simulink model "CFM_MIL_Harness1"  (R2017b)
settings: Solver=FixedStepDiscrete  StartTime=0.0  StopTime=14  FixedStep=0.01  RelTol=1e-3  EnableMultiTasking=on
undefined symbols (not defined in the file): sigbuilder_block
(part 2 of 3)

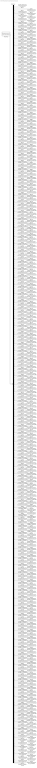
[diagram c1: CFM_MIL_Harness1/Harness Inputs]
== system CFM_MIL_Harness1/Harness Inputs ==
  Demux : Demux  Tag=STV Demux  Outputs=425
  FromWs : FromWorkspace  Tag=STV FromWs  VariableName=tuvar  SampleTime=0
  GaISP_AFEComLost_numb(1) : Outport  Tag=STV Outport
  GaISP_AFEComLost_numb(2) : Outport  Tag=STV Outport  Port=2
  GaISP_AFEComLost_numb(3) : Outport  Tag=STV Outport  Port=3
  GaISP_AFEComLost_numb(4) : Outport  Tag=STV Outport  Port=4
  GaISP_AFEComLost_numb(5) : Outport  Tag=STV Outport  Port=5
  GaISP_AFEComLost_numb(6) : Outport  Tag=STV Outport  Port=6
  GaISP_AFEComLost_numb(7) : Outport  Tag=STV Outport  Port=7
  GaISP_AFEComLost_numb(8) : Outport  Tag=STV Outport  Port=8
  GaISP_AFECellVoltUpdErr_numb(1) : Outport  Tag=STV Outport  Port=9
  GaISP_AFECellVoltUpdErr_numb(2) : Outport  Tag=STV Outport  Port=10
  GaISP_AFECellVoltUpdErr_numb(3) : Outport  Tag=STV Outport  Port=11
  GaISP_AFECellVoltUpdErr_numb(4) : Outport  Tag=STV Outport  Port=12
  GaISP_AFECellVoltUpdErr_numb(5) : Outport  Tag=STV Outport  Port=13
  GaISP_AFECellVoltUpdErr_numb(6) : Outport  Tag=STV Outport  Port=14
  GaISP_AFECellVoltUpdErr_numb(7) : Outport  Tag=STV Outport  Port=15
  GaISP_AFECellVoltUpdErr_numb(8) : Outport  Tag=STV Outport  Port=16
  GaISP_AFECellVoltUpdErr_numb(9) : Outport  Tag=STV Outport  Port=17
  GaISP_AFECellVoltUpdErr_numb(10) : Outport  Tag=STV Outport  Port=18
  GaISP_AFECellVoltUpdErr_numb(11) : Outport  Tag=STV Outport  Port=19
  GaISP_AFECellVoltUpdErr_numb(12) : Outport  Tag=STV Outport  Port=20
  GaISP_AFECellVoltUpdErr_numb(13) : Outport  Tag=STV Outport  Port=21
  GaISP_AFECellVoltUpdErr_numb(14) : Outport  Tag=STV Outport  Port=22
  GaISP_AFECellVoltUpdErr_numb(15) : Outport  Tag=STV Outport  Port=23
  GaISP_AFECellVoltUpdErr_numb(16) : Outport  Tag=STV Outport  Port=24
  GaISP_AFECellVoltUpdErr_numb(17) : Outport  Tag=STV Outport  Port=25
  GaISP_AFECellVoltUpdErr_numb(18) : Outport  Tag=STV Outport  Port=26
  GaISP_AFECellVoltUpdErr_numb(19) : Outport  Tag=STV Outport  Port=27
  GaISP_AFECellVoltUpdErr_numb(20) : Outport  Tag=STV Outport  Port=28
  GaISP_AFECellVoltUpdErr_numb(21) : Outport  Tag=STV Outport  Port=29
  GaISP_AFECellVoltUpdErr_numb(22) : Outport  Tag=STV Outport  Port=30
  GaISP_AFECellVoltUpdErr_numb(23) : Outport  Tag=STV Outport  Port=31
  GaISP_AFECellVoltUpdErr_numb(24) : Outport  Tag=STV Outport  Port=32
  GaISP_AFECellVoltUpdErr_numb(25) : Outport  Tag=STV Outport  Port=33
  GaISP_AFECellVoltUpdErr_numb(26) : Outport  Tag=STV Outport  Port=34
  GaISP_AFECellVoltUpdErr_numb(27) : Outport  Tag=STV Outport  Port=35
  GaISP_AFECellVoltUpdErr_numb(28) : Outport  Tag=STV Outport  Port=36
  GaISP_AFECellVoltUpdErr_numb(29) : Outport  Tag=STV Outport  Port=37
  GaISP_AFECellVoltUpdErr_numb(30) : Outport  Tag=STV Outport  Port=38
  GaISP_AFECellVoltUpdErr_numb(31) : Outport  Tag=STV Outport  Port=39
  GaISP_AFECellVoltUpdErr_numb(32) : Outport  Tag=STV Outport  Port=40
  GaISP_AFECellVoltUpdErr_numb(33) : Outport  Tag=STV Outport  Port=41
  GaISP_AFECellVoltUpdErr_numb(34) : Outport  Tag=STV Outport  Port=42
  GaISP_AFECellVoltUpdErr_numb(35) : Outport  Tag=STV Outport  Port=43
  GaISP_AFECellVoltUpdErr_numb(36) : Outport  Tag=STV Outport  Port=44
  GaISP_AFECellVoltUpdErr_numb(37) : Outport  Tag=STV Outport  Port=45
  GaISP_AFECellVoltUpdErr_numb(38) : Outport  Tag=STV Outport  Port=46
  GaISP_AFECellVoltUpdErr_numb(39) : Outport  Tag=STV Outport  Port=47
  GaISP_AFECellVoltUpdErr_numb(40) : Outport  Tag=STV Outport  Port=48
  GaISP_AFECellVoltUpdErr_numb(41) : Outport  Tag=STV Outport  Port=49
  GaISP_AFECellVoltUpdErr_numb(42) : Outport  Tag=STV Outport  Port=50
  GaISP_AFECellVoltUpdErr_numb(43) : Outport  Tag=STV Outport  Port=51
  GaISP_AFECellVoltUpdErr_numb(44) : Outport  Tag=STV Outport  Port=52
  GaISP_AFECellVoltUpdErr_numb(45) : Outport  Tag=STV Outport  Port=53
  GaISP_AFECellVoltUpdErr_numb(46) : Outport  Tag=STV Outport  Port=54
  GaISP_AFECellVoltUpdErr_numb(47) : Outport  Tag=STV Outport  Port=55
  GaISP_AFECellVoltUpdErr_numb(48) : Outport  Tag=STV Outport  Port=56
  GaISP_AFECellVoltUpdErr_numb(49) : Outport  Tag=STV Outport  Port=57
  GaISP_AFECellVoltUpdErr_numb(50) : Outport  Tag=STV Outport  Port=58
  GaISP_AFECellVoltUpdErr_numb(51) : Outport  Tag=STV Outport  Port=59
  GaISP_AFECellVoltUpdErr_numb(52) : Outport  Tag=STV Outport  Port=60
  GaISP_AFECellVoltUpdErr_numb(53) : Outport  Tag=STV Outport  Port=61
  GaISP_AFECellVoltUpdErr_numb(54) : Outport  Tag=STV Outport  Port=62
  GaISP_AFECellVoltUpdErr_numb(55) : Outport  Tag=STV Outport  Port=63
  GaISP_AFECellVoltUpdErr_numb(56) : Outport  Tag=STV Outport  Port=64
  GaISP_AFECellVoltUpdErr_numb(57) : Outport  Tag=STV Outport  Port=65
  GaISP_AFECellVoltUpdErr_numb(58) : Outport  Tag=STV Outport  Port=66
  GaISP_AFECellVoltUpdErr_numb(59) : Outport  Tag=STV Outport  Port=67
  GaISP_AFECellVoltUpdErr_numb(60) : Outport  Tag=STV Outport  Port=68
  GaISP_AFECellVoltUpdErr_numb(61) : Outport  Tag=STV Outport  Port=69
  GaISP_AFECellVoltUpdErr_numb(62) : Outport  Tag=STV Outport  Port=70
  GaISP_AFECellVoltUpdErr_numb(63) : Outport  Tag=STV Outport  Port=71
  GaISP_AFECellVoltUpdErr_numb(64) : Outport  Tag=STV Outport  Port=72
  GaISP_AFECellVoltUpdErr_numb(65) : Outport  Tag=STV Outport  Port=73
  GaISP_AFECellVoltUpdErr_numb(66) : Outport  Tag=STV Outport  Port=74
  GaISP_AFECellVoltUpdErr_numb(67) : Outport  Tag=STV Outport  Port=75
  GaISP_AFECellVoltUpdErr_numb(68) : Outport  Tag=STV Outport  Port=76
  GaISP_AFECellVoltUpdErr_numb(69) : Outport  Tag=STV Outport  Port=77
  GaISP_AFECellVoltUpdErr_numb(70) : Outport  Tag=STV Outport  Port=78
  GaISP_AFECellVoltUpdErr_numb(71) : Outport  Tag=STV Outport  Port=79
  GaISP_AFECellVoltUpdErr_numb(72) : Outport  Tag=STV Outport  Port=80
  GaISP_AFECellVoltUpdErr_numb(73) : Outport  Tag=STV Outport  Port=81
  GaISP_AFECellVoltUpdErr_numb(74) : Outport  Tag=STV Outport  Port=82
  GaISP_AFECellVoltUpdErr_numb(75) : Outport  Tag=STV Outport  Port=83
  GaISP_AFECellVoltUpdErr_numb(76) : Outport  Tag=STV Outport  Port=84
  GaISP_AFECellVoltUpdErr_numb(77) : Outport  Tag=STV Outport  Port=85
  GaISP_AFECellVoltUpdErr_numb(78) : Outport  Tag=STV Outport  Port=86
  GaISP_AFECellVoltUpdErr_numb(79) : Outport  Tag=STV Outport  Port=87
  GaISP_AFECellVoltUpdErr_numb(80) : Outport  Tag=STV Outport  Port=88
  GaISP_AFECellVoltUpdErr_numb(81) : Outport  Tag=STV Outport  Port=89
  GaISP_AFECellVoltUpdErr_numb(82) : Outport  Tag=STV Outport  Port=90
  GaISP_AFECellVoltUpdErr_numb(83) : Outport  Tag=STV Outport  Port=91
  GaISP_AFECellVoltUpdErr_numb(84) : Outport  Tag=STV Outport  Port=92
  GaISP_AFECellVoltUpdErr_numb(85) : Outport  Tag=STV Outport  Port=93
  GaISP_AFECellVoltUpdErr_numb(86) : Outport  Tag=STV Outport  Port=94
  GaISP_AFECellVoltUpdErr_numb(87) : Outport  Tag=STV Outport  Port=95
  GaISP_AFECellVoltUpdErr_numb(88) : Outport  Tag=STV Outport  Port=96
  GaISP_AFECellVoltUpdErr_numb(89) : Outport  Tag=STV Outport  Port=97
  GaISP_AFECellVoltUpdErr_numb(90) : Outport  Tag=STV Outport  Port=98
  GaISP_AFECellVoltUpdErr_numb(91) : Outport  Tag=STV Outport  Port=99
  GaISP_AFECellVoltUpdErr_numb(92) : Outport  Tag=STV Outport  Port=100
  GaISP_AFECellVoltUpdErr_numb(93) : Outport  Tag=STV Outport  Port=101
  GaISP_AFECellVoltUpdErr_numb(94) : Outport  Tag=STV Outport  Port=102
  GaISP_AFECellVoltUpdErr_numb(95) : Outport  Tag=STV Outport  Port=103
  GaISP_AFECellVoltUpdErr_numb(96) : Outport  Tag=STV Outport  Port=104
  GaISP_AFECellVoltUpdErr_numb(97) : Outport  Tag=STV Outport  Port=105
  GaISP_AFECellVoltUpdErr_numb(98) : Outport  Tag=STV Outport  Port=106
  GaISP_AFECellVoltUpdErr_numb(99) : Outport  Tag=STV Outport  Port=107
  GaISP_AFECellVoltUpdErr_numb(100) : Outport  Tag=STV Outport  Port=108
  GaISP_AFECellVoltUpdErr_numb(101) : Outport  Tag=STV Outport  Port=109
  GaISP_AFECellVoltUpdErr_numb(102) : Outport  Tag=STV Outport  Port=110
  GaISP_AFECellVoltUpdErr_numb(103) : Outport  Tag=STV Outport  Port=111
  GaISP_AFECellVoltUpdErr_numb(104) : Outport  Tag=STV Outport  Port=112
  GaISP_AFECellVoltUpdErr_numb(105) : Outport  Tag=STV Outport  Port=113
  GaISP_AFECellVoltUpdErr_numb(106) : Outport  Tag=STV Outport  Port=114
  GaISP_AFECellVoltUpdErr_numb(107) : Outport  Tag=STV Outport  Port=115
  GaISP_AFECellVoltUpdErr_numb(108) : Outport  Tag=STV Outport  Port=116
  GaISP_AFECellVoltUpdErr_numb(109) : Outport  Tag=STV Outport  Port=117
  GaISP_AFECellVoltUpdErr_numb(110) : Outport  Tag=STV Outport  Port=118
  GaISP_AFECellVoltUpdErr_numb(111) : Outport  Tag=STV Outport  Port=119
  GaISP_AFECellVoltUpdErr_numb(112) : Outport  Tag=STV Outport  Port=120
  GaISP_AFECellTempUpdErr_numb(1) : Outport  Tag=STV Outport  Port=121
  GaISP_AFECellTempUpdErr_numb(2) : Outport  Tag=STV Outport  Port=122
  GaISP_AFECellTempUpdErr_numb(3) : Outport  Tag=STV Outport  Port=123
  GaISP_AFECellTempUpdErr_numb(4) : Outport  Tag=STV Outport  Port=124
  GaISP_AFECellTempUpdErr_numb(5) : Outport  Tag=STV Outport  Port=125
  GaISP_AFECellTempUpdErr_numb(6) : Outport  Tag=STV Outport  Port=126
  GaISP_AFECellTempUpdErr_numb(7) : Outport  Tag=STV Outport  Port=127
  GaISP_AFECellTempUpdErr_numb(8) : Outport  Tag=STV Outport  Port=128
  GaISP_AFECellTempUpdErr_numb(9) : Outport  Tag=STV Outport  Port=129
  GaISP_AFECellTempUpdErr_numb(10) : Outport  Tag=STV Outport  Port=130
  GaISP_AFECellTempUpdErr_numb(11) : Outport  Tag=STV Outport  Port=131
  GaISP_AFECellTempUpdErr_numb(12) : Outport  Tag=STV Outport  Port=132
  GaISP_AFECellTempUpdErr_numb(13) : Outport  Tag=STV Outport  Port=133
  GaISP_AFECellTempUpdErr_numb(14) : Outport  Tag=STV Outport  Port=134
  GaISP_AFECellTempUpdErr_numb(15) : Outport  Tag=STV Outport  Port=135
  GaISP_AFECellTempUpdErr_numb(16) : Outport  Tag=STV Outport  Port=136
  GaISP_AFECellTempUpdErr_numb(17) : Outport  Tag=STV Outport  Port=137
  GaISP_AFECellTempUpdErr_numb(18) : Outport  Tag=STV Outport  Port=138
  GaISP_AFECellTempUpdErr_numb(19) : Outport  Tag=STV Outport  Port=139
  GaISP_AFECellTempUpdErr_numb(20) : Outport  Tag=STV Outport  Port=140
  GaISP_AFECellTempUpdErr_numb(21) : Outport  Tag=STV Outport  Port=141
  GaISP_AFECellTempUpdErr_numb(22) : Outport  Tag=STV Outport  Port=142
  GaISP_AFECellTempUpdErr_numb(23) : Outport  Tag=STV Outport  Port=143
  GaISP_AFECellTempUpdErr_numb(24) : Outport  Tag=STV Outport  Port=144
  GaISP_AFECellTempUpdErr_numb(25) : Outport  Tag=STV Outport  Port=145
  GaISP_AFECellTempUpdErr_numb(26) : Outport  Tag=STV Outport  Port=146
  GaISP_AFECellTempUpdErr_numb(27) : Outport  Tag=STV Outport  Port=147
  GaISP_AFECellTempUpdErr_numb(28) : Outport  Tag=STV Outport  Port=148
  GaISP_AFECellTempUpdErr_numb(29) : Outport  Tag=STV Outport  Port=149
  GaISP_AFECellTempUpdErr_numb(30) : Outport  Tag=STV Outport  Port=150
  GaISP_AFECellTempUpdErr_numb(31) : Outport  Tag=STV Outport  Port=151
  GaISP_AFECellTempUpdErr_numb(32) : Outport  Tag=STV Outport  Port=152
  GaISP_AFECellTempUpdErr_numb(33) : Outport  Tag=STV Outport  Port=153
  GaISP_AFECellTempUpdErr_numb(34) : Outport  Tag=STV Outport  Port=154
  GaISP_AFECellTempUpdErr_numb(35) : Outport  Tag=STV Outport  Port=155
  GaISP_AFECellTempUpdErr_numb(36) : Outport  Tag=STV Outport  Port=156
  GaISP_AFECellTempUpdErr_numb(37) : Outport  Tag=STV Outport  Port=157
  GaISP_AFECellTempUpdErr_numb(38) : Outport  Tag=STV Outport  Port=158
  GaISP_AFECellTempUpdErr_numb(39) : Outport  Tag=STV Outport  Port=159
  GaISP_AFECellTempUpdErr_numb(40) : Outport  Tag=STV Outport  Port=160
  GaISP_AFECellTempUpdErr_numb(41) : Outport  Tag=STV Outport  Port=161
  GaISP_AFECellTempUpdErr_numb(42) : Outport  Tag=STV Outport  Port=162
  GaISP_AFECellTempUpdErr_numb(43) : Outport  Tag=STV Outport  Port=163
  GaISP_AFECellTempUpdErr_numb(44) : Outport  Tag=STV Outport  Port=164
  GaISP_AFECellTempUpdErr_numb(45) : Outport  Tag=STV Outport  Port=165
  GaISP_AFECellTempUpdErr_numb(46) : Outport  Tag=STV Outport  Port=166
  GaISP_AFECellTempUpdErr_numb(47) : Outport  Tag=STV Outport  Port=167
  GaISP_AFECellTempUpdErr_numb(48) : Outport  Tag=STV Outport  Port=168
  GaISP_AFECellVoltLineOpen_numb(1) : Outport  Tag=STV Outport  Port=169
  GaISP_AFECellVoltLineOpen_numb(2) : Outport  Tag=STV Outport  Port=170
  GaISP_AFECellVoltLineOpen_numb(3) : Outport  Tag=STV Outport  Port=171
  GaISP_AFECellVoltLineOpen_numb(4) : Outport  Tag=STV Outport  Port=172
  GaISP_AFECellVoltLineOpen_numb(5) : Outport  Tag=STV Outport  Port=173
  GaISP_AFECellVoltLineOpen_numb(6) : Outport  Tag=STV Outport  Port=174
  GaISP_AFECellVoltLineOpen_numb(7) : Outport  Tag=STV Outport  Port=175
  GaISP_AFECellVoltLineOpen_numb(8) : Outport  Tag=STV Outport  Port=176
  GaISP_AFECellVoltLineOpen_numb(9) : Outport  Tag=STV Outport  Port=177
  GaISP_AFECellVoltLineOpen_numb(10) : Outport  Tag=STV Outport  Port=178
  GaISP_AFECellVoltLineOpen_numb(11) : Outport  Tag=STV Outport  Port=179
  GaISP_AFECellVoltLineOpen_numb(12) : Outport  Tag=STV Outport  Port=180
  GaISP_AFECellVoltLineOpen_numb(13) : Outport  Tag=STV Outport  Port=181
  GaISP_AFECellVoltLineOpen_numb(14) : Outport  Tag=STV Outport  Port=182
  GaISP_AFECellVoltLineOpen_numb(15) : Outport  Tag=STV Outport  Port=183
  GaISP_AFECellVoltLineOpen_numb(16) : Outport  Tag=STV Outport  Port=184
  GaISP_AFECellVoltLineOpen_numb(17) : Outport  Tag=STV Outport  Port=185
  GaISP_AFECellVoltLineOpen_numb(18) : Outport  Tag=STV Outport  Port=186
  GaISP_AFECellVoltLineOpen_numb(19) : Outport  Tag=STV Outport  Port=187
  GaISP_AFECellVoltLineOpen_numb(20) : Outport  Tag=STV Outport  Port=188
  GaISP_AFECellVoltLineOpen_numb(21) : Outport  Tag=STV Outport  Port=189
  GaISP_AFECellVoltLineOpen_numb(22) : Outport  Tag=STV Outport  Port=190
  GaISP_AFECellVoltLineOpen_numb(23) : Outport  Tag=STV Outport  Port=191
  GaISP_AFECellVoltLineOpen_numb(24) : Outport  Tag=STV Outport  Port=192
  GaISP_AFECellVoltLineOpen_numb(25) : Outport  Tag=STV Outport  Port=193
  GaISP_AFECellVoltLineOpen_numb(26) : Outport  Tag=STV Outport  Port=194
  GaISP_AFECellVoltLineOpen_numb(27) : Outport  Tag=STV Outport  Port=195
  GaISP_AFECellVoltLineOpen_numb(28) : Outport  Tag=STV Outport  Port=196
  GaISP_AFECellVoltLineOpen_numb(29) : Outport  Tag=STV Outport  Port=197
  GaISP_AFECellVoltLineOpen_numb(30) : Outport  Tag=STV Outport  Port=198
  GaISP_AFECellVoltLineOpen_numb(31) : Outport  Tag=STV Outport  Port=199
  GaISP_AFECellVoltLineOpen_numb(32) : Outport  Tag=STV Outport  Port=200
  GaISP_AFECellVoltLineOpen_numb(33) : Outport  Tag=STV Outport  Port=201
  GaISP_AFECellVoltLineOpen_numb(34) : Outport  Tag=STV Outport  Port=202
  GaISP_AFECellVoltLineOpen_numb(35) : Outport  Tag=STV Outport  Port=203
  GaISP_AFECellVoltLineOpen_numb(36) : Outport  Tag=STV Outport  Port=204
  GaISP_AFECellVoltLineOpen_numb(37) : Outport  Tag=STV Outport  Port=205
  GaISP_AFECellVoltLineOpen_numb(38) : Outport  Tag=STV Outport  Port=206
  GaISP_AFECellVoltLineOpen_numb(39) : Outport  Tag=STV Outport  Port=207
  GaISP_AFECellVoltLineOpen_numb(40) : Outport  Tag=STV Outport  Port=208
  GaISP_AFECellVoltLineOpen_numb(41) : Outport  Tag=STV Outport  Port=209
  GaISP_AFECellVoltLineOpen_numb(42) : Outport  Tag=STV Outport  Port=210
  GaISP_AFECellVoltLineOpen_numb(43) : Outport  Tag=STV Outport  Port=211
  GaISP_AFECellVoltLineOpen_numb(44) : Outport  Tag=STV Outport  Port=212
  GaISP_AFECellVoltLineOpen_numb(45) : Outport  Tag=STV Outport  Port=213
  GaISP_AFECellVoltLineOpen_numb(46) : Outport  Tag=STV Outport  Port=214
  GaISP_AFECellVoltLineOpen_numb(47) : Outport  Tag=STV Outport  Port=215
  GaISP_AFECellVoltLineOpen_numb(48) : Outport  Tag=STV Outport  Port=216
  GaISP_AFECellVoltLineOpen_numb(49) : Outport  Tag=STV Outport  Port=217
  GaISP_AFECellVoltLineOpen_numb(50) : Outport  Tag=STV Outport  Port=218
  GaISP_AFECellVoltLineOpen_numb(51) : Outport  Tag=STV Outport  Port=219
  GaISP_AFECellVoltLineOpen_numb(52) : Outport  Tag=STV Outport  Port=220
  GaISP_AFECellVoltLineOpen_numb(53) : Outport  Tag=STV Outport  Port=221
  GaISP_AFECellVoltLineOpen_numb(54) : Outport  Tag=STV Outport  Port=222
  GaISP_AFECellVoltLineOpen_numb(55) : Outport  Tag=STV Outport  Port=223
  GaISP_AFECellVoltLineOpen_numb(56) : Outport  Tag=STV Outport  Port=224
  GaISP_AFECellVoltLineOpen_numb(57) : Outport  Tag=STV Outport  Port=225
  GaISP_AFECellVoltLineOpen_numb(58) : Outport  Tag=STV Outport  Port=226
  GaISP_AFECellVoltLineOpen_numb(59) : Outport  Tag=STV Outport  Port=227
  GaISP_AFECellVoltLineOpen_numb(60) : Outport  Tag=STV Outport  Port=228
  GaISP_AFECellVoltLineOpen_numb(61) : Outport  Tag=STV Outport  Port=229
  GaISP_AFECellVoltLineOpen_numb(62) : Outport  Tag=STV Outport  Port=230
  GaISP_AFECellVoltLineOpen_numb(63) : Outport  Tag=STV Outport  Port=231
  GaISP_AFECellVoltLineOpen_numb(64) : Outport  Tag=STV Outport  Port=232
  GaISP_AFECellVoltLineOpen_numb(65) : Outport  Tag=STV Outport  Port=233
  GaISP_AFECellVoltLineOpen_numb(66) : Outport  Tag=STV Outport  Port=234
  GaISP_AFECellVoltLineOpen_numb(67) : Outport  Tag=STV Outport  Port=235
  GaISP_AFECellVoltLineOpen_numb(68) : Outport  Tag=STV Outport  Port=236
  GaISP_AFECellVoltLineOpen_numb(69) : Outport  Tag=STV Outport  Port=237
  GaISP_AFECellVoltLineOpen_numb(70) : Outport  Tag=STV Outport  Port=238
  GaISP_AFECellVoltLineOpen_numb(71) : Outport  Tag=STV Outport  Port=239
  GaISP_AFECellVoltLineOpen_numb(72) : Outport  Tag=STV Outport  Port=240
  GaISP_AFECellVoltLineOpen_numb(73) : Outport  Tag=STV Outport  Port=241
  GaISP_AFECellVoltLineOpen_numb(74) : Outport  Tag=STV Outport  Port=242
  GaISP_AFECellVoltLineOpen_numb(75) : Outport  Tag=STV Outport  Port=243
  GaISP_AFECellVoltLineOpen_numb(76) : Outport  Tag=STV Outport  Port=244
  GaISP_AFECellVoltLineOpen_numb(77) : Outport  Tag=STV Outport  Port=245
  GaISP_AFECellVoltLineOpen_numb(78) : Outport  Tag=STV Outport  Port=246
  GaISP_AFECellVoltLineOpen_numb(79) : Outport  Tag=STV Outport  Port=247
  GaISP_AFECellVoltLineOpen_numb(80) : Outport  Tag=STV Outport  Port=248
  GaISP_AFECellVoltLineOpen_numb(81) : Outport  Tag=STV Outport  Port=249
  GaISP_AFECellVoltLineOpen_numb(82) : Outport  Tag=STV Outport  Port=250
  GaISP_AFECellVoltLineOpen_numb(83) : Outport  Tag=STV Outport  Port=251
  GaISP_AFECellVoltLineOpen_numb(84) : Outport  Tag=STV Outport  Port=252
  GaISP_AFECellVoltLineOpen_numb(85) : Outport  Tag=STV Outport  Port=253
  GaISP_AFECellVoltLineOpen_numb(86) : Outport  Tag=STV Outport  Port=254
  GaISP_AFECellVoltLineOpen_numb(87) : Outport  Tag=STV Outport  Port=255
  GaISP_AFECellVoltLineOpen_numb(88) : Outport  Tag=STV Outport  Port=256
  GaISP_AFECellVoltLineOpen_numb(89) : Outport  Tag=STV Outport  Port=257
  GaISP_AFECellVoltLineOpen_numb(90) : Outport  Tag=STV Outport  Port=258
  GaISP_AFECellVoltLineOpen_numb(91) : Outport  Tag=STV Outport  Port=259
  GaISP_AFECellVoltLineOpen_numb(92) : Outport  Tag=STV Outport  Port=260
  GaISP_AFECellVoltLineOpen_numb(93) : Outport  Tag=STV Outport  Port=261
  GaISP_AFECellVoltLineOpen_numb(94) : Outport  Tag=STV Outport  Port=262
  GaISP_AFECellVoltLineOpen_numb(95) : Outport  Tag=STV Outport  Port=263
  GaISP_AFECellVoltLineOpen_numb(96) : Outport  Tag=STV Outport  Port=264
  GaISP_AFECellVoltLineOpen_numb(97) : Outport  Tag=STV Outport  Port=265
  GaISP_AFECellVoltLineOpen_numb(98) : Outport  Tag=STV Outport  Port=266
  GaISP_AFECellVoltLineOpen_numb(99) : Outport  Tag=STV Outport  Port=267
  GaISP_AFECellVoltLineOpen_numb(100) : Outport  Tag=STV Outport  Port=268
  GaISP_AFECellVoltLineOpen_numb(101) : Outport  Tag=STV Outport  Port=269
  GaISP_AFECellVoltLineOpen_numb(102) : Outport  Tag=STV Outport  Port=270
  GaISP_AFECellVoltLineOpen_numb(103) : Outport  Tag=STV Outport  Port=271
  GaISP_AFECellVoltLineOpen_numb(104) : Outport  Tag=STV Outport  Port=272
  GaISP_AFECellVoltLineOpen_numb(105) : Outport  Tag=STV Outport  Port=273
  GaISP_AFECellVoltLineOpen_numb(106) : Outport  Tag=STV Outport  Port=274
  GaISP_AFECellVoltLineOpen_numb(107) : Outport  Tag=STV Outport  Port=275
  GaISP_AFECellVoltLineOpen_numb(108) : Outport  Tag=STV Outport  Port=276
  GaISP_AFECellVoltLineOpen_numb(109) : Outport  Tag=STV Outport  Port=277
  GaISP_AFECellVoltLineOpen_numb(110) : Outport  Tag=STV Outport  Port=278
  GaISP_AFECellVoltLineOpen_numb(111) : Outport  Tag=STV Outport  Port=279
  GaISP_AFECellVoltLineOpen_numb(112) : Outport  Tag=STV Outport  Port=280
  GaCDP_AFETempSampAbn_flg(1) : Outport  Tag=STV Outport  Port=281
  GaCDP_AFETempSampAbn_flg(2) : Outport  Tag=STV Outport  Port=282
  GaCDP_AFETempSampAbn_flg(3) : Outport  Tag=STV Outport  Port=283
  GaCDP_AFETempSampAbn_flg(4) : Outport  Tag=STV Outport  Port=284
  GaCDP_AFETempSampAbn_flg(5) : Outport  Tag=STV Outport  Port=285
  GaCDP_AFETempSampAbn_flg(6) : Outport  Tag=STV Outport  Port=286
  GaCDP_AFETempSampAbn_flg(7) : Outport  Tag=STV Outport  Port=287
  GaCDP_AFETempSampAbn_flg(8) : Outport  Tag=STV Outport  Port=288
  GaISP_AFEAdcRelatedErr_numb(1) : Outport  Tag=STV Outport  Port=289
  GaISP_AFEAdcRelatedErr_numb(2) : Outport  Tag=STV Outport  Port=290
  GaISP_AFEAdcRelatedErr_numb(3) : Outport  Tag=STV Outport  Port=291
  GaISP_AFEAdcRelatedErr_numb(4) : Outport  Tag=STV Outport  Port=292
  GaISP_AFEAdcRelatedErr_numb(5) : Outport  Tag=STV Outport  Port=293
  GaISP_AFEAdcRelatedErr_numb(6) : Outport  Tag=STV Outport  Port=294
  GaISP_AFEAdcRelatedErr_numb(7) : Outport  Tag=STV Outport  Port=295
  GaISP_AFEAdcRelatedErr_numb(8) : Outport  Tag=STV Outport  Port=296
  GaISP_AFEAdcRelatedErr_numb(9) : Outport  Tag=STV Outport  Port=297
  GaISP_AFEAdcRelatedErr_numb(10) : Outport  Tag=STV Outport  Port=298
  GaISP_AFEAdcRelatedErr_numb(11) : Outport  Tag=STV Outport  Port=299
  GaISP_AFEAdcRelatedErr_numb(12) : Outport  Tag=STV Outport  Port=300
  GaISP_AFEAdcRelatedErr_numb(13) : Outport  Tag=STV Outport  Port=301
  GaISP_AFEAdcRelatedErr_numb(14) : Outport  Tag=STV Outport  Port=302
  GaISP_AFEAdcRelatedErr_numb(15) : Outport  Tag=STV Outport  Port=303
  GaISP_AFEAdcRelatedErr_numb(16) : Outport  Tag=STV Outport  Port=304
  GaISP_AFEAdcRelatedErr_numb(17) : Outport  Tag=STV Outport  Port=305
  GaISP_AFEAdcRelatedErr_numb(18) : Outport  Tag=STV Outport  Port=306
  GaISP_AFEAdcRelatedErr_numb(19) : Outport  Tag=STV Outport  Port=307
  GaISP_AFEAdcRelatedErr_numb(20) : Outport  Tag=STV Outport  Port=308
  GaISP_AFEAdcRelatedErr_numb(21) : Outport  Tag=STV Outport  Port=309
  GaISP_AFEAdcRelatedErr_numb(22) : Outport  Tag=STV Outport  Port=310
  GaISP_AFEAdcRelatedErr_numb(23) : Outport  Tag=STV Outport  Port=311
  GaISP_AFEAdcRelatedErr_numb(24) : Outport  Tag=STV Outport  Port=312
  GaISP_AFEAdcRelatedErr_numb(25) : Outport  Tag=STV Outport  Port=313
  GaISP_AFEAdcRelatedErr_numb(26) : Outport  Tag=STV Outport  Port=314
  GaISP_AFEAdcRelatedErr_numb(27) : Outport  Tag=STV Outport  Port=315
  GaISP_AFEAdcRelatedErr_numb(28) : Outport  Tag=STV Outport  Port=316
  GaISP_AFEAdcRelatedErr_numb(29) : Outport  Tag=STV Outport  Port=317
  GaISP_AFEAdcRelatedErr_numb(30) : Outport  Tag=STV Outport  Port=318
  GaISP_AFEAdcRelatedErr_numb(31) : Outport  Tag=STV Outport  Port=319
  GaISP_AFEAdcRelatedErr_numb(32) : Outport  Tag=STV Outport  Port=320
  GaISP_AFEAdcRelatedErr_numb(33) : Outport  Tag=STV Outport  Port=321
  GaISP_AFEAdcRelatedErr_numb(34) : Outport  Tag=STV Outport  Port=322
  GaISP_AFEAdcRelatedErr_numb(35) : Outport  Tag=STV Outport  Port=323
  GaISP_AFEAdcRelatedErr_numb(36) : Outport  Tag=STV Outport  Port=324
  GaISP_AFEAdcRelatedErr_numb(37) : Outport  Tag=STV Outport  Port=325
  GaISP_AFEAdcRelatedErr_numb(38) : Outport  Tag=STV Outport  Port=326
  GaISP_AFEAdcRelatedErr_numb(39) : Outport  Tag=STV Outport  Port=327
  GaISP_AFEAdcRelatedErr_numb(40) : Outport  Tag=STV Outport  Port=328
  GaISP_AFEAdcRelatedErr_numb(41) : Outport  Tag=STV Outport  Port=329
  GaISP_AFEAdcRelatedErr_numb(42) : Outport  Tag=STV Outport  Port=330
  GaISP_AFEAdcRelatedErr_numb(43) : Outport  Tag=STV Outport  Port=331
  GaISP_AFEAdcRelatedErr_numb(44) : Outport  Tag=STV Outport  Port=332
  GaISP_AFEAdcRelatedErr_numb(45) : Outport  Tag=STV Outport  Port=333
  GaISP_AFEAdcRelatedErr_numb(46) : Outport  Tag=STV Outport  Port=334
  GaISP_AFEAdcRelatedErr_numb(47) : Outport  Tag=STV Outport  Port=335
  GaISP_AFEAdcRelatedErr_numb(48) : Outport  Tag=STV Outport  Port=336
  GaISP_AFEAdcRelatedErr_numb(49) : Outport  Tag=STV Outport  Port=337
  GaISP_AFEAdcRelatedErr_numb(50) : Outport  Tag=STV Outport  Port=338
  GaISP_AFEAdcRelatedErr_numb(51) : Outport  Tag=STV Outport  Port=339
  GaISP_AFEAdcRelatedErr_numb(52) : Outport  Tag=STV Outport  Port=340
  GaISP_AFEAdcRelatedErr_numb(53) : Outport  Tag=STV Outport  Port=341
  GaISP_AFEAdcRelatedErr_numb(54) : Outport  Tag=STV Outport  Port=342
  GaISP_AFEAdcRelatedErr_numb(55) : Outport  Tag=STV Outport  Port=343
  GaISP_AFEAdcRelatedErr_numb(56) : Outport  Tag=STV Outport  Port=344
  GaISP_AFEAdcRelatedErr_numb(57) : Outport  Tag=STV Outport  Port=345
  GaISP_AFEAdcRelatedErr_numb(58) : Outport  Tag=STV Outport  Port=346
  GaISP_AFEAdcRelatedErr_numb(59) : Outport  Tag=STV Outport  Port=347
  GaISP_AFEAdcRelatedErr_numb(60) : Outport  Tag=STV Outport  Port=348
  GaISP_AFEAdcRelatedErr_numb(61) : Outport  Tag=STV Outport  Port=349
  GaISP_AFEAdcRelatedErr_numb(62) : Outport  Tag=STV Outport  Port=350
  GaISP_AFEAdcRelatedErr_numb(63) : Outport  Tag=STV Outport  Port=351
  GaISP_AFEAdcRelatedErr_numb(64) : Outport  Tag=STV Outport  Port=352
  GaISP_AFEAdcRelatedErr_numb(65) : Outport  Tag=STV Outport  Port=353
  GaISP_AFEAdcRelatedErr_numb(66) : Outport  Tag=STV Outport  Port=354
  GaISP_AFEAdcRelatedErr_numb(67) : Outport  Tag=STV Outport  Port=355
  GaISP_AFEAdcRelatedErr_numb(68) : Outport  Tag=STV Outport  Port=356
  GaISP_AFEAdcRelatedErr_numb(69) : Outport  Tag=STV Outport  Port=357
  GaISP_AFEAdcRelatedErr_numb(70) : Outport  Tag=STV Outport  Port=358
  GaISP_AFEAdcRelatedErr_numb(71) : Outport  Tag=STV Outport  Port=359
  GaISP_AFEAdcRelatedErr_numb(72) : Outport  Tag=STV Outport  Port=360
  GaISP_AFEAdcRelatedErr_numb(73) : Outport  Tag=STV Outport  Port=361
  GaISP_AFEAdcRelatedErr_numb(74) : Outport  Tag=STV Outport  Port=362
  GaISP_AFEAdcRelatedErr_numb(75) : Outport  Tag=STV Outport  Port=363
  GaISP_AFEAdcRelatedErr_numb(76) : Outport  Tag=STV Outport  Port=364
  GaISP_AFEAdcRelatedErr_numb(77) : Outport  Tag=STV Outport  Port=365
  GaISP_AFEAdcRelatedErr_numb(78) : Outport  Tag=STV Outport  Port=366
  GaISP_AFEAdcRelatedErr_numb(79) : Outport  Tag=STV Outport  Port=367
  GaISP_AFEAdcRelatedErr_numb(80) : Outport  Tag=STV Outport  Port=368
  GaISP_AFEAdcRelatedErr_numb(81) : Outport  Tag=STV Outport  Port=369
  GaISP_AFEAdcRelatedErr_numb(82) : Outport  Tag=STV Outport  Port=370
  GaISP_AFEAdcRelatedErr_numb(83) : Outport  Tag=STV Outport  Port=371
  GaISP_AFEAdcRelatedErr_numb(84) : Outport  Tag=STV Outport  Port=372
  GaISP_AFEAdcRelatedErr_numb(85) : Outport  Tag=STV Outport  Port=373
  GaISP_AFEAdcRelatedErr_numb(86) : Outport  Tag=STV Outport  Port=374
  GaISP_AFEAdcRelatedErr_numb(87) : Outport  Tag=STV Outport  Port=375
  GaISP_AFEAdcRelatedErr_numb(88) : Outport  Tag=STV Outport  Port=376
  GaISP_AFEAdcRelatedErr_numb(89) : Outport  Tag=STV Outport  Port=377
  GaISP_AFEAdcRelatedErr_numb(90) : Outport  Tag=STV Outport  Port=378
  GaISP_AFEAdcRelatedErr_numb(91) : Outport  Tag=STV Outport  Port=379
  GaISP_AFEAdcRelatedErr_numb(92) : Outport  Tag=STV Outport  Port=380
  GaISP_AFEAdcRelatedErr_numb(93) : Outport  Tag=STV Outport  Port=381
  GaISP_AFEAdcRelatedErr_numb(94) : Outport  Tag=STV Outport  Port=382
  GaISP_AFEAdcRelatedErr_numb(95) : Outport  Tag=STV Outport  Port=383
  GaISP_AFEAdcRelatedErr_numb(96) : Outport  Tag=STV Outport  Port=384
  GaISP_AFEAdcRelatedErr_numb(97) : Outport  Tag=STV Outport  Port=385
  GaISP_AFEAdcRelatedErr_numb(98) : Outport  Tag=STV Outport  Port=386
  GaISP_AFEAdcRelatedErr_numb(99) : Outport  Tag=STV Outport  Port=387
  GaISP_AFEAdcRelatedErr_numb(100) : Outport  Tag=STV Outport  Port=388
  GaISP_AFEAdcRelatedErr_numb(101) : Outport  Tag=STV Outport  Port=389
  GaISP_AFEAdcRelatedErr_numb(102) : Outport  Tag=STV Outport  Port=390
  GaISP_AFEAdcRelatedErr_numb(103) : Outport  Tag=STV Outport  Port=391
  GaISP_AFEAdcRelatedErr_numb(104) : Outport  Tag=STV Outport  Port=392
  GaISP_AFEAdcRelatedErr_numb(105) : Outport  Tag=STV Outport  Port=393
  GaISP_AFEAdcRelatedErr_numb(106) : Outport  Tag=STV Outport  Port=394
  GaISP_AFEAdcRelatedErr_numb(107) : Outport  Tag=STV Outport  Port=395
  GaISP_AFEAdcRelatedErr_numb(108) : Outport  Tag=STV Outport  Port=396
  GaISP_AFEAdcRelatedErr_numb(109) : Outport  Tag=STV Outport  Port=397
  GaISP_AFEAdcRelatedErr_numb(110) : Outport  Tag=STV Outport  Port=398
  GaISP_AFEAdcRelatedErr_numb(111) : Outport  Tag=STV Outport  Port=399
  GaISP_AFEAdcRelatedErr_numb(112) : Outport  Tag=STV Outport  Port=400
  GaISP_AFEDiagModeExitErr_numb(1) : Outport  Tag=STV Outport  Port=401
  GaISP_AFEDiagModeExitErr_numb(2) : Outport  Tag=STV Outport  Port=402
  GaISP_AFEDiagModeExitErr_numb(3) : Outport  Tag=STV Outport  Port=403
  GaISP_AFEDiagModeExitErr_numb(4) : Outport  Tag=STV Outport  Port=404
  GaISP_AFEDiagModeExitErr_numb(5) : Outport  Tag=STV Outport  Port=405
  GaISP_AFEDiagModeExitErr_numb(6) : Outport  Tag=STV Outport  Port=406
  GaISP_AFEDiagModeExitErr_numb(7) : Outport  Tag=STV Outport  Port=407
  GaISP_AFEDiagModeExitErr_numb(8) : Outport  Tag=STV Outport  Port=408
  GaISP_AFEOtherErr_numb(1) : Outport  Tag=STV Outport  Port=409
  GaISP_AFEOtherErr_numb(2) : Outport  Tag=STV Outport  Port=410
  GaISP_AFEOtherErr_numb(3) : Outport  Tag=STV Outport  Port=411
  GaISP_AFEOtherErr_numb(4) : Outport  Tag=STV Outport  Port=412
  GaISP_AFEOtherErr_numb(5) : Outport  Tag=STV Outport  Port=413
  GaISP_AFEOtherErr_numb(6) : Outport  Tag=STV Outport  Port=414
  GaISP_AFEOtherErr_numb(7) : Outport  Tag=STV Outport  Port=415
  GaISP_AFEOtherErr_numb(8) : Outport  Tag=STV Outport  Port=416
  GaISP_AFESampleErr_numb(1) : Outport  Tag=STV Outport  Port=417
  GaISP_AFESampleErr_numb(2) : Outport  Tag=STV Outport  Port=418
  GaISP_AFESampleErr_numb(3) : Outport  Tag=STV Outport  Port=419
  GaISP_AFESampleErr_numb(4) : Outport  Tag=STV Outport  Port=420
  GaISP_AFESampleErr_numb(5) : Outport  Tag=STV Outport  Port=421
  GaISP_AFESampleErr_numb(6) : Outport  Tag=STV Outport  Port=422
  GaISP_AFESampleErr_numb(7) : Outport  Tag=STV Outport  Port=423
  GaISP_AFESampleErr_numb(8) : Outport  Tag=STV Outport  Port=424
  GeUDS_CapSel_enum : Outport  Tag=STV Outport  Port=425
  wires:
  FromWs/1 -> Demux/1
  Demux/1 -> GaISP_AFEComLost_numb(1)/1
  Demux/2 -> GaISP_AFEComLost_numb(2)/1
  Demux/3 -> GaISP_AFEComLost_numb(3)/1
  Demux/4 -> GaISP_AFEComLost_numb(4)/1
  Demux/5 -> GaISP_AFEComLost_numb(5)/1
  Demux/6 -> GaISP_AFEComLost_numb(6)/1
  Demux/7 -> GaISP_AFEComLost_numb(7)/1
  Demux/8 -> GaISP_AFEComLost_numb(8)/1
  Demux/9 -> GaISP_AFECellVoltUpdErr_numb(1)/1
  Demux/10 -> GaISP_AFECellVoltUpdErr_numb(2)/1
  Demux/11 -> GaISP_AFECellVoltUpdErr_numb(3)/1
  Demux/12 -> GaISP_AFECellVoltUpdErr_numb(4)/1
  Demux/13 -> GaISP_AFECellVoltUpdErr_numb(5)/1
  Demux/14 -> GaISP_AFECellVoltUpdErr_numb(6)/1
  Demux/15 -> GaISP_AFECellVoltUpdErr_numb(7)/1
  Demux/16 -> GaISP_AFECellVoltUpdErr_numb(8)/1
  Demux/17 -> GaISP_AFECellVoltUpdErr_numb(9)/1
  Demux/18 -> GaISP_AFECellVoltUpdErr_numb(10)/1
  Demux/19 -> GaISP_AFECellVoltUpdErr_numb(11)/1
  Demux/20 -> GaISP_AFECellVoltUpdErr_numb(12)/1
  Demux/21 -> GaISP_AFECellVoltUpdErr_numb(13)/1
  Demux/22 -> GaISP_AFECellVoltUpdErr_numb(14)/1
  Demux/23 -> GaISP_AFECellVoltUpdErr_numb(15)/1
  Demux/24 -> GaISP_AFECellVoltUpdErr_numb(16)/1
  Demux/25 -> GaISP_AFECellVoltUpdErr_numb(17)/1
  Demux/26 -> GaISP_AFECellVoltUpdErr_numb(18)/1
  Demux/27 -> GaISP_AFECellVoltUpdErr_numb(19)/1
  Demux/28 -> GaISP_AFECellVoltUpdErr_numb(20)/1
  Demux/29 -> GaISP_AFECellVoltUpdErr_numb(21)/1
  Demux/30 -> GaISP_AFECellVoltUpdErr_numb(22)/1
  Demux/31 -> GaISP_AFECellVoltUpdErr_numb(23)/1
  Demux/32 -> GaISP_AFECellVoltUpdErr_numb(24)/1
  Demux/33 -> GaISP_AFECellVoltUpdErr_numb(25)/1
  Demux/34 -> GaISP_AFECellVoltUpdErr_numb(26)/1
  Demux/35 -> GaISP_AFECellVoltUpdErr_numb(27)/1
  Demux/36 -> GaISP_AFECellVoltUpdErr_numb(28)/1
  Demux/37 -> GaISP_AFECellVoltUpdErr_numb(29)/1
  Demux/38 -> GaISP_AFECellVoltUpdErr_numb(30)/1
  Demux/39 -> GaISP_AFECellVoltUpdErr_numb(31)/1
  Demux/40 -> GaISP_AFECellVoltUpdErr_numb(32)/1
  Demux/41 -> GaISP_AFECellVoltUpdErr_numb(33)/1
  Demux/42 -> GaISP_AFECellVoltUpdErr_numb(34)/1
  Demux/43 -> GaISP_AFECellVoltUpdErr_numb(35)/1
  Demux/44 -> GaISP_AFECellVoltUpdErr_numb(36)/1
  Demux/45 -> GaISP_AFECellVoltUpdErr_numb(37)/1
  Demux/46 -> GaISP_AFECellVoltUpdErr_numb(38)/1
  Demux/47 -> GaISP_AFECellVoltUpdErr_numb(39)/1
  Demux/48 -> GaISP_AFECellVoltUpdErr_numb(40)/1
  Demux/49 -> GaISP_AFECellVoltUpdErr_numb(41)/1
  Demux/50 -> GaISP_AFECellVoltUpdErr_numb(42)/1
  Demux/51 -> GaISP_AFECellVoltUpdErr_numb(43)/1
  Demux/52 -> GaISP_AFECellVoltUpdErr_numb(44)/1
  Demux/53 -> GaISP_AFECellVoltUpdErr_numb(45)/1
  Demux/54 -> GaISP_AFECellVoltUpdErr_numb(46)/1
  Demux/55 -> GaISP_AFECellVoltUpdErr_numb(47)/1
  Demux/56 -> GaISP_AFECellVoltUpdErr_numb(48)/1
  Demux/57 -> GaISP_AFECellVoltUpdErr_numb(49)/1
  Demux/58 -> GaISP_AFECellVoltUpdErr_numb(50)/1
  Demux/59 -> GaISP_AFECellVoltUpdErr_numb(51)/1
  Demux/60 -> GaISP_AFECellVoltUpdErr_numb(52)/1
  Demux/61 -> GaISP_AFECellVoltUpdErr_numb(53)/1
  Demux/62 -> GaISP_AFECellVoltUpdErr_numb(54)/1
  Demux/63 -> GaISP_AFECellVoltUpdErr_numb(55)/1
  Demux/64 -> GaISP_AFECellVoltUpdErr_numb(56)/1
  Demux/65 -> GaISP_AFECellVoltUpdErr_numb(57)/1
  Demux/66 -> GaISP_AFECellVoltUpdErr_numb(58)/1
  Demux/67 -> GaISP_AFECellVoltUpdErr_numb(59)/1
  Demux/68 -> GaISP_AFECellVoltUpdErr_numb(60)/1
  Demux/69 -> GaISP_AFECellVoltUpdErr_numb(61)/1
  Demux/70 -> GaISP_AFECellVoltUpdErr_numb(62)/1
  Demux/71 -> GaISP_AFECellVoltUpdErr_numb(63)/1
  Demux/72 -> GaISP_AFECellVoltUpdErr_numb(64)/1
  Demux/73 -> GaISP_AFECellVoltUpdErr_numb(65)/1
  Demux/74 -> GaISP_AFECellVoltUpdErr_numb(66)/1
  Demux/75 -> GaISP_AFECellVoltUpdErr_numb(67)/1
  Demux/76 -> GaISP_AFECellVoltUpdErr_numb(68)/1
  Demux/77 -> GaISP_AFECellVoltUpdErr_numb(69)/1
  Demux/78 -> GaISP_AFECellVoltUpdErr_numb(70)/1
  Demux/79 -> GaISP_AFECellVoltUpdErr_numb(71)/1
  Demux/80 -> GaISP_AFECellVoltUpdErr_numb(72)/1
  Demux/81 -> GaISP_AFECellVoltUpdErr_numb(73)/1
  Demux/82 -> GaISP_AFECellVoltUpdErr_numb(74)/1
  Demux/83 -> GaISP_AFECellVoltUpdErr_numb(75)/1
  Demux/84 -> GaISP_AFECellVoltUpdErr_numb(76)/1
  Demux/85 -> GaISP_AFECellVoltUpdErr_numb(77)/1
  Demux/86 -> GaISP_AFECellVoltUpdErr_numb(78)/1
  Demux/87 -> GaISP_AFECellVoltUpdErr_numb(79)/1
  Demux/88 -> GaISP_AFECellVoltUpdErr_numb(80)/1
  Demux/89 -> GaISP_AFECellVoltUpdErr_numb(81)/1
  Demux/90 -> GaISP_AFECellVoltUpdErr_numb(82)/1
  Demux/91 -> GaISP_AFECellVoltUpdErr_numb(83)/1
  Demux/92 -> GaISP_AFECellVoltUpdErr_numb(84)/1
  Demux/93 -> GaISP_AFECellVoltUpdErr_numb(85)/1
  Demux/94 -> GaISP_AFECellVoltUpdErr_numb(86)/1
  Demux/95 -> GaISP_AFECellVoltUpdErr_numb(87)/1
  Demux/96 -> GaISP_AFECellVoltUpdErr_numb(88)/1
  Demux/97 -> GaISP_AFECellVoltUpdErr_numb(89)/1
  Demux/98 -> GaISP_AFECellVoltUpdErr_numb(90)/1
  Demux/99 -> GaISP_AFECellVoltUpdErr_numb(91)/1
  Demux/100 -> GaISP_AFECellVoltUpdErr_numb(92)/1
  Demux/101 -> GaISP_AFECellVoltUpdErr_numb(93)/1
  Demux/102 -> GaISP_AFECellVoltUpdErr_numb(94)/1
  Demux/103 -> GaISP_AFECellVoltUpdErr_numb(95)/1
  Demux/104 -> GaISP_AFECellVoltUpdErr_numb(96)/1
  Demux/105 -> GaISP_AFECellVoltUpdErr_numb(97)/1
  Demux/106 -> GaISP_AFECellVoltUpdErr_numb(98)/1
  Demux/107 -> GaISP_AFECellVoltUpdErr_numb(99)/1
  Demux/108 -> GaISP_AFECellVoltUpdErr_numb(100)/1
  Demux/109 -> GaISP_AFECellVoltUpdErr_numb(101)/1
  Demux/110 -> GaISP_AFECellVoltUpdErr_numb(102)/1
  Demux/111 -> GaISP_AFECellVoltUpdErr_numb(103)/1
  Demux/112 -> GaISP_AFECellVoltUpdErr_numb(104)/1
  Demux/113 -> GaISP_AFECellVoltUpdErr_numb(105)/1
  Demux/114 -> GaISP_AFECellVoltUpdErr_numb(106)/1
  Demux/115 -> GaISP_AFECellVoltUpdErr_numb(107)/1
  Demux/116 -> GaISP_AFECellVoltUpdErr_numb(108)/1
  Demux/117 -> GaISP_AFECellVoltUpdErr_numb(109)/1
  Demux/118 -> GaISP_AFECellVoltUpdErr_numb(110)/1
  Demux/119 -> GaISP_AFECellVoltUpdErr_numb(111)/1
  Demux/120 -> GaISP_AFECellVoltUpdErr_numb(112)/1
  Demux/121 -> GaISP_AFECellTempUpdErr_numb(1)/1
  Demux/122 -> GaISP_AFECellTempUpdErr_numb(2)/1
  Demux/123 -> GaISP_AFECellTempUpdErr_numb(3)/1
  Demux/124 -> GaISP_AFECellTempUpdErr_numb(4)/1
  Demux/125 -> GaISP_AFECellTempUpdErr_numb(5)/1
  Demux/126 -> GaISP_AFECellTempUpdErr_numb(6)/1
  Demux/127 -> GaISP_AFECellTempUpdErr_numb(7)/1
  Demux/128 -> GaISP_AFECellTempUpdErr_numb(8)/1
  Demux/129 -> GaISP_AFECellTempUpdErr_numb(9)/1
  Demux/130 -> GaISP_AFECellTempUpdErr_numb(10)/1
  Demux/131 -> GaISP_AFECellTempUpdErr_numb(11)/1
  Demux/132 -> GaISP_AFECellTempUpdErr_numb(12)/1
  Demux/133 -> GaISP_AFECellTempUpdErr_numb(13)/1
  Demux/134 -> GaISP_AFECellTempUpdErr_numb(14)/1
  Demux/135 -> GaISP_AFECellTempUpdErr_numb(15)/1
  Demux/136 -> GaISP_AFECellTempUpdErr_numb(16)/1
  Demux/137 -> GaISP_AFECellTempUpdErr_numb(17)/1
  Demux/138 -> GaISP_AFECellTempUpdErr_numb(18)/1
  Demux/139 -> GaISP_AFECellTempUpdErr_numb(19)/1
  Demux/140 -> GaISP_AFECellTempUpdErr_numb(20)/1
  Demux/141 -> GaISP_AFECellTempUpdErr_numb(21)/1
  Demux/142 -> GaISP_AFECellTempUpdErr_numb(22)/1
  Demux/143 -> GaISP_AFECellTempUpdErr_numb(23)/1
  Demux/144 -> GaISP_AFECellTempUpdErr_numb(24)/1
  Demux/145 -> GaISP_AFECellTempUpdErr_numb(25)/1
  Demux/146 -> GaISP_AFECellTempUpdErr_numb(26)/1
  Demux/147 -> GaISP_AFECellTempUpdErr_numb(27)/1
  Demux/148 -> GaISP_AFECellTempUpdErr_numb(28)/1
  Demux/149 -> GaISP_AFECellTempUpdErr_numb(29)/1
  Demux/150 -> GaISP_AFECellTempUpdErr_numb(30)/1
  Demux/151 -> GaISP_AFECellTempUpdErr_numb(31)/1
  Demux/152 -> GaISP_AFECellTempUpdErr_numb(32)/1
  Demux/153 -> GaISP_AFECellTempUpdErr_numb(33)/1
  Demux/154 -> GaISP_AFECellTempUpdErr_numb(34)/1
  Demux/155 -> GaISP_AFECellTempUpdErr_numb(35)/1
  Demux/156 -> GaISP_AFECellTempUpdErr_numb(36)/1
  Demux/157 -> GaISP_AFECellTempUpdErr_numb(37)/1
  Demux/158 -> GaISP_AFECellTempUpdErr_numb(38)/1
  Demux/159 -> GaISP_AFECellTempUpdErr_numb(39)/1
  Demux/160 -> GaISP_AFECellTempUpdErr_numb(40)/1
  Demux/161 -> GaISP_AFECellTempUpdErr_numb(41)/1
  Demux/162 -> GaISP_AFECellTempUpdErr_numb(42)/1
  Demux/163 -> GaISP_AFECellTempUpdErr_numb(43)/1
  Demux/164 -> GaISP_AFECellTempUpdErr_numb(44)/1
  Demux/165 -> GaISP_AFECellTempUpdErr_numb(45)/1
  Demux/166 -> GaISP_AFECellTempUpdErr_numb(46)/1
  Demux/167 -> GaISP_AFECellTempUpdErr_numb(47)/1
  Demux/168 -> GaISP_AFECellTempUpdErr_numb(48)/1
  Demux/169 -> GaISP_AFECellVoltLineOpen_numb(1)/1
  Demux/170 -> GaISP_AFECellVoltLineOpen_numb(2)/1
  Demux/171 -> GaISP_AFECellVoltLineOpen_numb(3)/1
  Demux/172 -> GaISP_AFECellVoltLineOpen_numb(4)/1
  Demux/173 -> GaISP_AFECellVoltLineOpen_numb(5)/1
  Demux/174 -> GaISP_AFECellVoltLineOpen_numb(6)/1
  Demux/175 -> GaISP_AFECellVoltLineOpen_numb(7)/1
  Demux/176 -> GaISP_AFECellVoltLineOpen_numb(8)/1
  Demux/177 -> GaISP_AFECellVoltLineOpen_numb(9)/1
  Demux/178 -> GaISP_AFECellVoltLineOpen_numb(10)/1
  Demux/179 -> GaISP_AFECellVoltLineOpen_numb(11)/1
  Demux/180 -> GaISP_AFECellVoltLineOpen_numb(12)/1
  Demux/181 -> GaISP_AFECellVoltLineOpen_numb(13)/1
  Demux/182 -> GaISP_AFECellVoltLineOpen_numb(14)/1
  Demux/183 -> GaISP_AFECellVoltLineOpen_numb(15)/1
  Demux/184 -> GaISP_AFECellVoltLineOpen_numb(16)/1
  Demux/185 -> GaISP_AFECellVoltLineOpen_numb(17)/1
  Demux/186 -> GaISP_AFECellVoltLineOpen_numb(18)/1
  Demux/187 -> GaISP_AFECellVoltLineOpen_numb(19)/1
  Demux/188 -> GaISP_AFECellVoltLineOpen_numb(20)/1
  Demux/189 -> GaISP_AFECellVoltLineOpen_numb(21)/1
  Demux/190 -> GaISP_AFECellVoltLineOpen_numb(22)/1
  Demux/191 -> GaISP_AFECellVoltLineOpen_numb(23)/1
  Demux/192 -> GaISP_AFECellVoltLineOpen_numb(24)/1
  Demux/193 -> GaISP_AFECellVoltLineOpen_numb(25)/1
  Demux/194 -> GaISP_AFECellVoltLineOpen_numb(26)/1
  Demux/195 -> GaISP_AFECellVoltLineOpen_numb(27)/1
  Demux/196 -> GaISP_AFECellVoltLineOpen_numb(28)/1
  Demux/197 -> GaISP_AFECellVoltLineOpen_numb(29)/1
  Demux/198 -> GaISP_AFECellVoltLineOpen_numb(30)/1
  Demux/199 -> GaISP_AFECellVoltLineOpen_numb(31)/1
  Demux/200 -> GaISP_AFECellVoltLineOpen_numb(32)/1
  Demux/201 -> GaISP_AFECellVoltLineOpen_numb(33)/1
  Demux/202 -> GaISP_AFECellVoltLineOpen_numb(34)/1
  Demux/203 -> GaISP_AFECellVoltLineOpen_numb(35)/1
  Demux/204 -> GaISP_AFECellVoltLineOpen_numb(36)/1
  Demux/205 -> GaISP_AFECellVoltLineOpen_numb(37)/1
  Demux/206 -> GaISP_AFECellVoltLineOpen_numb(38)/1
  Demux/207 -> GaISP_AFECellVoltLineOpen_numb(39)/1
  Demux/208 -> GaISP_AFECellVoltLineOpen_numb(40)/1
  Demux/209 -> GaISP_AFECellVoltLineOpen_numb(41)/1
  Demux/210 -> GaISP_AFECellVoltLineOpen_numb(42)/1
  Demux/211 -> GaISP_AFECellVoltLineOpen_numb(43)/1
  Demux/212 -> GaISP_AFECellVoltLineOpen_numb(44)/1
  Demux/213 -> GaISP_AFECellVoltLineOpen_numb(45)/1
  Demux/214 -> GaISP_AFECellVoltLineOpen_numb(46)/1
  Demux/215 -> GaISP_AFECellVoltLineOpen_numb(47)/1
  Demux/216 -> GaISP_AFECellVoltLineOpen_numb(48)/1
  Demux/217 -> GaISP_AFECellVoltLineOpen_numb(49)/1
  Demux/218 -> GaISP_AFECellVoltLineOpen_numb(50)/1
  Demux/219 -> GaISP_AFECellVoltLineOpen_numb(51)/1
  Demux/220 -> GaISP_AFECellVoltLineOpen_numb(52)/1
  Demux/221 -> GaISP_AFECellVoltLineOpen_numb(53)/1
  Demux/222 -> GaISP_AFECellVoltLineOpen_numb(54)/1
  Demux/223 -> GaISP_AFECellVoltLineOpen_numb(55)/1
  Demux/224 -> GaISP_AFECellVoltLineOpen_numb(56)/1
  Demux/225 -> GaISP_AFECellVoltLineOpen_numb(57)/1
  Demux/226 -> GaISP_AFECellVoltLineOpen_numb(58)/1
  Demux/227 -> GaISP_AFECellVoltLineOpen_numb(59)/1
  Demux/228 -> GaISP_AFECellVoltLineOpen_numb(60)/1
  Demux/229 -> GaISP_AFECellVoltLineOpen_numb(61)/1
  Demux/230 -> GaISP_AFECellVoltLineOpen_numb(62)/1
  Demux/231 -> GaISP_AFECellVoltLineOpen_numb(63)/1
  Demux/232 -> GaISP_AFECellVoltLineOpen_numb(64)/1
  Demux/233 -> GaISP_AFECellVoltLineOpen_numb(65)/1
  Demux/234 -> GaISP_AFECellVoltLineOpen_numb(66)/1
  Demux/235 -> GaISP_AFECellVoltLineOpen_numb(67)/1
  Demux/236 -> GaISP_AFECellVoltLineOpen_numb(68)/1
  Demux/237 -> GaISP_AFECellVoltLineOpen_numb(69)/1
  Demux/238 -> GaISP_AFECellVoltLineOpen_numb(70)/1
  Demux/239 -> GaISP_AFECellVoltLineOpen_numb(71)/1
  Demux/240 -> GaISP_AFECellVoltLineOpen_numb(72)/1
  Demux/241 -> GaISP_AFECellVoltLineOpen_numb(73)/1
  Demux/242 -> GaISP_AFECellVoltLineOpen_numb(74)/1
  Demux/243 -> GaISP_AFECellVoltLineOpen_numb(75)/1
  Demux/244 -> GaISP_AFECellVoltLineOpen_numb(76)/1
  Demux/245 -> GaISP_AFECellVoltLineOpen_numb(77)/1
  Demux/246 -> GaISP_AFECellVoltLineOpen_numb(78)/1
  Demux/247 -> GaISP_AFECellVoltLineOpen_numb(79)/1
  Demux/248 -> GaISP_AFECellVoltLineOpen_numb(80)/1
  Demux/249 -> GaISP_AFECellVoltLineOpen_numb(81)/1
  Demux/250 -> GaISP_AFECellVoltLineOpen_numb(82)/1
  Demux/251 -> GaISP_AFECellVoltLineOpen_numb(83)/1
  Demux/252 -> GaISP_AFECellVoltLineOpen_numb(84)/1
  Demux/253 -> GaISP_AFECellVoltLineOpen_numb(85)/1
  Demux/254 -> GaISP_AFECellVoltLineOpen_numb(86)/1
  Demux/255 -> GaISP_AFECellVoltLineOpen_numb(87)/1
  Demux/256 -> GaISP_AFECellVoltLineOpen_numb(88)/1
  Demux/257 -> GaISP_AFECellVoltLineOpen_numb(89)/1
  Demux/258 -> GaISP_AFECellVoltLineOpen_numb(90)/1
  Demux/259 -> GaISP_AFECellVoltLineOpen_numb(91)/1
  Demux/260 -> GaISP_AFECellVoltLineOpen_numb(92)/1
  Demux/261 -> GaISP_AFECellVoltLineOpen_numb(93)/1
  Demux/262 -> GaISP_AFECellVoltLineOpen_numb(94)/1
  Demux/263 -> GaISP_AFECellVoltLineOpen_numb(95)/1
  Demux/264 -> GaISP_AFECellVoltLineOpen_numb(96)/1
  Demux/265 -> GaISP_AFECellVoltLineOpen_numb(97)/1
  Demux/266 -> GaISP_AFECellVoltLineOpen_numb(98)/1
  Demux/267 -> GaISP_AFECellVoltLineOpen_numb(99)/1
  Demux/268 -> GaISP_AFECellVoltLineOpen_numb(100)/1
  Demux/269 -> GaISP_AFECellVoltLineOpen_numb(101)/1
  Demux/270 -> GaISP_AFECellVoltLineOpen_numb(102)/1
  Demux/271 -> GaISP_AFECellVoltLineOpen_numb(103)/1
  Demux/272 -> GaISP_AFECellVoltLineOpen_numb(104)/1
  Demux/273 -> GaISP_AFECellVoltLineOpen_numb(105)/1
  Demux/274 -> GaISP_AFECellVoltLineOpen_numb(106)/1
  Demux/275 -> GaISP_AFECellVoltLineOpen_numb(107)/1
  Demux/276 -> GaISP_AFECellVoltLineOpen_numb(108)/1
  Demux/277 -> GaISP_AFECellVoltLineOpen_numb(109)/1
  Demux/278 -> GaISP_AFECellVoltLineOpen_numb(110)/1
  Demux/279 -> GaISP_AFECellVoltLineOpen_numb(111)/1
  Demux/280 -> GaISP_AFECellVoltLineOpen_numb(112)/1
  Demux/281 -> GaCDP_AFETempSampAbn_flg(1)/1
  Demux/282 -> GaCDP_AFETempSampAbn_flg(2)/1
  Demux/283 -> GaCDP_AFETempSampAbn_flg(3)/1
  Demux/284 -> GaCDP_AFETempSampAbn_flg(4)/1
  Demux/285 -> GaCDP_AFETempSampAbn_flg(5)/1
  Demux/286 -> GaCDP_AFETempSampAbn_flg(6)/1
  Demux/287 -> GaCDP_AFETempSampAbn_flg(7)/1
  Demux/288 -> GaCDP_AFETempSampAbn_flg(8)/1
  Demux/289 -> GaISP_AFEAdcRelatedErr_numb(1)/1
  Demux/290 -> GaISP_AFEAdcRelatedErr_numb(2)/1
  Demux/291 -> GaISP_AFEAdcRelatedErr_numb(3)/1
  Demux/292 -> GaISP_AFEAdcRelatedErr_numb(4)/1
  Demux/293 -> GaISP_AFEAdcRelatedErr_numb(5)/1
  Demux/294 -> GaISP_AFEAdcRelatedErr_numb(6)/1
  Demux/295 -> GaISP_AFEAdcRelatedErr_numb(7)/1
  Demux/296 -> GaISP_AFEAdcRelatedErr_numb(8)/1
  Demux/297 -> GaISP_AFEAdcRelatedErr_numb(9)/1
  Demux/298 -> GaISP_AFEAdcRelatedErr_numb(10)/1
  Demux/299 -> GaISP_AFEAdcRelatedErr_numb(11)/1
  Demux/300 -> GaISP_AFEAdcRelatedErr_numb(12)/1
  Demux/301 -> GaISP_AFEAdcRelatedErr_numb(13)/1
  Demux/302 -> GaISP_AFEAdcRelatedErr_numb(14)/1
  Demux/303 -> GaISP_AFEAdcRelatedErr_numb(15)/1
  Demux/304 -> GaISP_AFEAdcRelatedErr_numb(16)/1
  Demux/305 -> GaISP_AFEAdcRelatedErr_numb(17)/1
  Demux/306 -> GaISP_AFEAdcRelatedErr_numb(18)/1
  Demux/307 -> GaISP_AFEAdcRelatedErr_numb(19)/1
  Demux/308 -> GaISP_AFEAdcRelatedErr_numb(20)/1
  Demux/309 -> GaISP_AFEAdcRelatedErr_numb(21)/1
  Demux/310 -> GaISP_AFEAdcRelatedErr_numb(22)/1
  Demux/311 -> GaISP_AFEAdcRelatedErr_numb(23)/1
  Demux/312 -> GaISP_AFEAdcRelatedErr_numb(24)/1
  Demux/313 -> GaISP_AFEAdcRelatedErr_numb(25)/1
  Demux/314 -> GaISP_AFEAdcRelatedErr_numb(26)/1
  Demux/315 -> GaISP_AFEAdcRelatedErr_numb(27)/1
  Demux/316 -> GaISP_AFEAdcRelatedErr_numb(28)/1
  Demux/317 -> GaISP_AFEAdcRelatedErr_numb(29)/1
  Demux/318 -> GaISP_AFEAdcRelatedErr_numb(30)/1
  Demux/319 -> GaISP_AFEAdcRelatedErr_numb(31)/1
  Demux/320 -> GaISP_AFEAdcRelatedErr_numb(32)/1
  Demux/321 -> GaISP_AFEAdcRelatedErr_numb(33)/1
  Demux/322 -> GaISP_AFEAdcRelatedErr_numb(34)/1
  Demux/323 -> GaISP_AFEAdcRelatedErr_numb(35)/1
  Demux/324 -> GaISP_AFEAdcRelatedErr_numb(36)/1
  Demux/325 -> GaISP_AFEAdcRelatedErr_numb(37)/1
  Demux/326 -> GaISP_AFEAdcRelatedErr_numb(38)/1
  Demux/327 -> GaISP_AFEAdcRelatedErr_numb(39)/1
  Demux/328 -> GaISP_AFEAdcRelatedErr_numb(40)/1
  Demux/329 -> GaISP_AFEAdcRelatedErr_numb(41)/1
  Demux/330 -> GaISP_AFEAdcRelatedErr_numb(42)/1
  Demux/331 -> GaISP_AFEAdcRelatedErr_numb(43)/1
  Demux/332 -> GaISP_AFEAdcRelatedErr_numb(44)/1
  Demux/333 -> GaISP_AFEAdcRelatedErr_numb(45)/1
  Demux/334 -> GaISP_AFEAdcRelatedErr_numb(46)/1
  Demux/335 -> GaISP_AFEAdcRelatedErr_numb(47)/1
  Demux/336 -> GaISP_AFEAdcRelatedErr_numb(48)/1
  Demux/337 -> GaISP_AFEAdcRelatedErr_numb(49)/1
  Demux/338 -> GaISP_AFEAdcRelatedErr_numb(50)/1
  Demux/339 -> GaISP_AFEAdcRelatedErr_numb(51)/1
  Demux/340 -> GaISP_AFEAdcRelatedErr_numb(52)/1
  Demux/341 -> GaISP_AFEAdcRelatedErr_numb(53)/1
  Demux/342 -> GaISP_AFEAdcRelatedErr_numb(54)/1
  Demux/343 -> GaISP_AFEAdcRelatedErr_numb(55)/1
  Demux/344 -> GaISP_AFEAdcRelatedErr_numb(56)/1
  Demux/345 -> GaISP_AFEAdcRelatedErr_numb(57)/1
  Demux/346 -> GaISP_AFEAdcRelatedErr_numb(58)/1
  Demux/347 -> GaISP_AFEAdcRelatedErr_numb(59)/1
  Demux/348 -> GaISP_AFEAdcRelatedErr_numb(60)/1
  Demux/349 -> GaISP_AFEAdcRelatedErr_numb(61)/1
  Demux/350 -> GaISP_AFEAdcRelatedErr_numb(62)/1
  Demux/351 -> GaISP_AFEAdcRelatedErr_numb(63)/1
  Demux/352 -> GaISP_AFEAdcRelatedErr_numb(64)/1
  Demux/353 -> GaISP_AFEAdcRelatedErr_numb(65)/1
  Demux/354 -> GaISP_AFEAdcRelatedErr_numb(66)/1
  Demux/355 -> GaISP_AFEAdcRelatedErr_numb(67)/1
  Demux/356 -> GaISP_AFEAdcRelatedErr_numb(68)/1
  Demux/357 -> GaISP_AFEAdcRelatedErr_numb(69)/1
  Demux/358 -> GaISP_AFEAdcRelatedErr_numb(70)/1
  Demux/359 -> GaISP_AFEAdcRelatedErr_numb(71)/1
  Demux/360 -> GaISP_AFEAdcRelatedErr_numb(72)/1
  Demux/361 -> GaISP_AFEAdcRelatedErr_numb(73)/1
  Demux/362 -> GaISP_AFEAdcRelatedErr_numb(74)/1
  Demux/363 -> GaISP_AFEAdcRelatedErr_numb(75)/1
  Demux/364 -> GaISP_AFEAdcRelatedErr_numb(76)/1
  Demux/365 -> GaISP_AFEAdcRelatedErr_numb(77)/1
  Demux/366 -> GaISP_AFEAdcRelatedErr_numb(78)/1
  Demux/367 -> GaISP_AFEAdcRelatedErr_numb(79)/1
  Demux/368 -> GaISP_AFEAdcRelatedErr_numb(80)/1
  Demux/369 -> GaISP_AFEAdcRelatedErr_numb(81)/1
  Demux/370 -> GaISP_AFEAdcRelatedErr_numb(82)/1
  Demux/371 -> GaISP_AFEAdcRelatedErr_numb(83)/1
  Demux/372 -> GaISP_AFEAdcRelatedErr_numb(84)/1
  Demux/373 -> GaISP_AFEAdcRelatedErr_numb(85)/1
  Demux/374 -> GaISP_AFEAdcRelatedErr_numb(86)/1
  Demux/375 -> GaISP_AFEAdcRelatedErr_numb(87)/1
  Demux/376 -> GaISP_AFEAdcRelatedErr_numb(88)/1
  Demux/377 -> GaISP_AFEAdcRelatedErr_numb(89)/1
  Demux/378 -> GaISP_AFEAdcRelatedErr_numb(90)/1
  Demux/379 -> GaISP_AFEAdcRelatedErr_numb(91)/1
  Demux/380 -> GaISP_AFEAdcRelatedErr_numb(92)/1
  Demux/381 -> GaISP_AFEAdcRelatedErr_numb(93)/1
  Demux/382 -> GaISP_AFEAdcRelatedErr_numb(94)/1
  Demux/383 -> GaISP_AFEAdcRelatedErr_numb(95)/1
  Demux/384 -> GaISP_AFEAdcRelatedErr_numb(96)/1
  Demux/385 -> GaISP_AFEAdcRelatedErr_numb(97)/1
  Demux/386 -> GaISP_AFEAdcRelatedErr_numb(98)/1
  Demux/387 -> GaISP_AFEAdcRelatedErr_numb(99)/1
  Demux/388 -> GaISP_AFEAdcRelatedErr_numb(100)/1
  Demux/389 -> GaISP_AFEAdcRelatedErr_numb(101)/1
  Demux/390 -> GaISP_AFEAdcRelatedErr_numb(102)/1
  Demux/391 -> GaISP_AFEAdcRelatedErr_numb(103)/1
  Demux/392 -> GaISP_AFEAdcRelatedErr_numb(104)/1
  Demux/393 -> GaISP_AFEAdcRelatedErr_numb(105)/1
  Demux/394 -> GaISP_AFEAdcRelatedErr_numb(106)/1
  Demux/395 -> GaISP_AFEAdcRelatedErr_numb(107)/1
  Demux/396 -> GaISP_AFEAdcRelatedErr_numb(108)/1
  Demux/397 -> GaISP_AFEAdcRelatedErr_numb(109)/1
  Demux/398 -> GaISP_AFEAdcRelatedErr_numb(110)/1
  Demux/399 -> GaISP_AFEAdcRelatedErr_numb(111)/1
  Demux/400 -> GaISP_AFEAdcRelatedErr_numb(112)/1
  Demux/401 -> GaISP_AFEDiagModeExitErr_numb(1)/1
  Demux/402 -> GaISP_AFEDiagModeExitErr_numb(2)/1
  Demux/403 -> GaISP_AFEDiagModeExitErr_numb(3)/1
  Demux/404 -> GaISP_AFEDiagModeExitErr_numb(4)/1
  Demux/405 -> GaISP_AFEDiagModeExitErr_numb(5)/1
  Demux/406 -> GaISP_AFEDiagModeExitErr_numb(6)/1
  Demux/407 -> GaISP_AFEDiagModeExitErr_numb(7)/1
  Demux/408 -> GaISP_AFEDiagModeExitErr_numb(8)/1
  Demux/409 -> GaISP_AFEOtherErr_numb(1)/1
  Demux/410 -> GaISP_AFEOtherErr_numb(2)/1
  Demux/411 -> GaISP_AFEOtherErr_numb(3)/1
  Demux/412 -> GaISP_AFEOtherErr_numb(4)/1
  Demux/413 -> GaISP_AFEOtherErr_numb(5)/1
  Demux/414 -> GaISP_AFEOtherErr_numb(6)/1
  Demux/415 -> GaISP_AFEOtherErr_numb(7)/1
  Demux/416 -> GaISP_AFEOtherErr_numb(8)/1
  Demux/417 -> GaISP_AFESampleErr_numb(1)/1
  Demux/418 -> GaISP_AFESampleErr_numb(2)/1
  Demux/419 -> GaISP_AFESampleErr_numb(3)/1
  Demux/420 -> GaISP_AFESampleErr_numb(4)/1
  Demux/421 -> GaISP_AFESampleErr_numb(5)/1
  Demux/422 -> GaISP_AFESampleErr_numb(6)/1
  Demux/423 -> GaISP_AFESampleErr_numb(7)/1
  Demux/424 -> GaISP_AFESampleErr_numb(8)/1
  Demux/425 -> GeUDS_CapSel_enum/1
